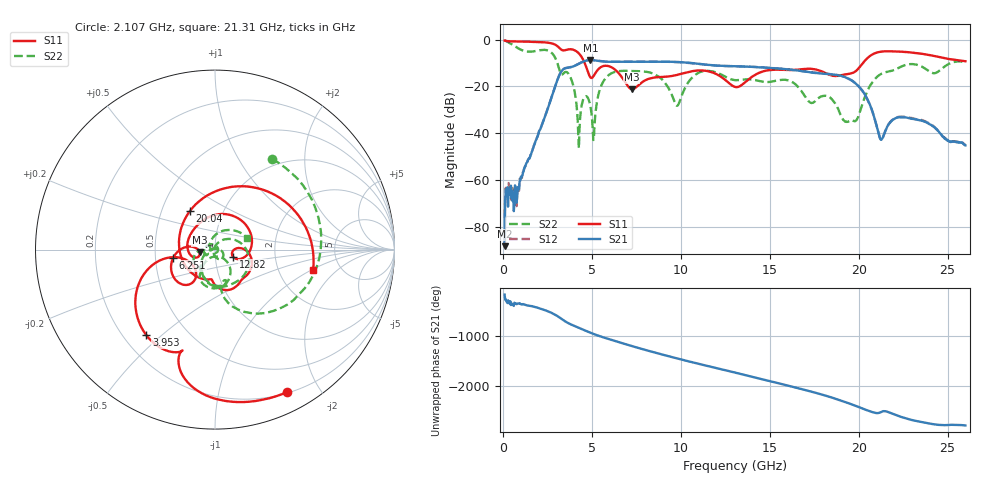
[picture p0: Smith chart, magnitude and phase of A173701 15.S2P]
!  2-Port S-parameters saved by WinCal
! VAR MeasName=S-Parameters (CALIBRATED_DATA) read from VNA (N5245A)
! VAR MeasDate=2017-6-7 10:29:21
! VAR NAME=A173701 15
! VAR FILENAME=A173701 15.S2P
! VAR DATE=2017-6-7 10:29:21
! VAR PHYS_PORTS=1,2
# Hz S DB R 50
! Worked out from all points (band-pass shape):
!   801 points, 100 MHz to 26 GHz, reference 50 ohm
!   highest |S21| = -8.71 dB at 4.924 GHz (marker M1); lowest = -88.4 dB at 100 MHz (marker M2)
!   |S21| within 3 dB of the highest: 3.84 GHz to 14.26 GHz (10.42 GHz wide, 115 % of centre)
!   lowest |S11| = -21.2 dB at 7.255 GHz (marker M3), VSWR 1.19, Z = 42.1 - j1.31 ohm
!   |S11| at or under -10 dB: 4.601 GHz to 20.24 GHz (15.64 GHz wide, 126 % of centre)
!   |S22| runs from -46.5 to -0.3 dB; largest |S21 - S12| = 0.0047
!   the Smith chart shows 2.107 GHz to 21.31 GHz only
!   S11 on the Smith chart (normalised r, x): 2.107 GHz: 0.21, -1.61; 3.953 GHz: 0.29, -0.45; 6.251 GHz: 0.62, -0.06; 12.82 GHz: 1.22, -0.10; 20.04 GHz: 0.69, +0.32; 21.31 GHz: 3.16, -1.03
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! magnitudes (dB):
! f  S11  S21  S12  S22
! 100 MHz  -0.3  -88.4  -76.1  -0.3
! 2.107 GHz  -1.0  -38.3  -38.3  -4.5
! 3.208 GHz  -3.7  -14.7  -14.6  -13.6
! 3.953 GHz  -4.3  -11.4  -11.4  -19.5
! 4.244 GHz  -5.6  -10.4  -10.4  -41.5
! 4.438 GHz  -7.5  -9.6  -9.6  -27.8
! 4.924 GHz  -16.1  -8.7  -8.7  -28.5
! 5.118 GHz  -15.3  -8.8  -8.8  -42.4
! 5.539 GHz  -11.6  -9.2  -9.2  -19.6
! 6.251 GHz  -12.5  -9.5  -9.5  -13.9
! 7.255 GHz  -21.2  -9.4  -9.4  -13.4
! 8.744 GHz  -16.0  -9.4  -9.4  -15.7
! 9.78 GHz  -15.1  -9.5  -9.6  -28.3
! 11.04 GHz  -13.1  -10.3  -10.4  -14.0
! 12.82 GHz  -19.2  -11.3  -11.3  -16.9
! 13.05 GHz  -20.2  -11.4  -11.4  -17.3
! 16.06 GHz  -13.0  -12.7  -12.7  -17.4
! 17.39 GHz  -12.5  -14.1  -13.9  -27.0
! 20.04 GHz  -11.8  -20.3  -20.3  -31.4
! 21.31 GHz  -5.1  -42.5  -42.6  -14.5
! 21.69 GHz  -4.9  -36.1  -35.9  -13.6
! 26 GHz  -9.2  -45.2  -45.3  -9.9
